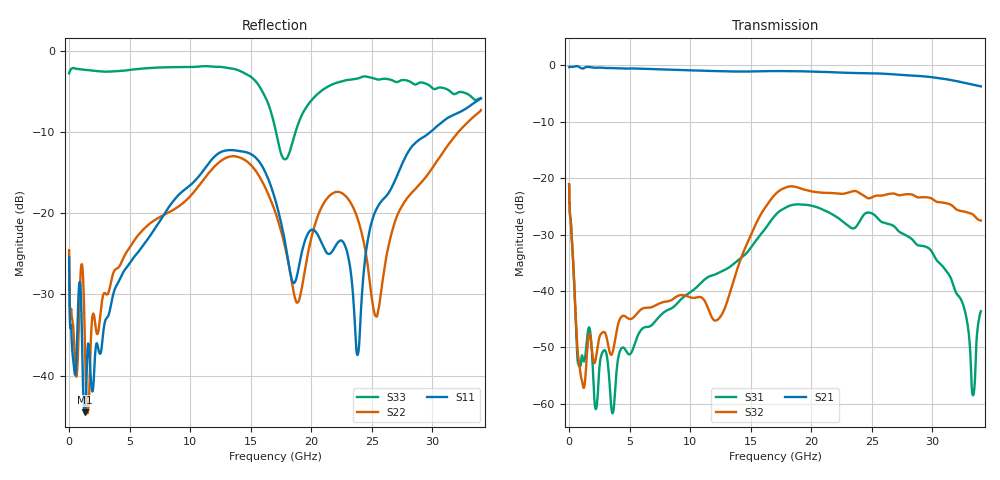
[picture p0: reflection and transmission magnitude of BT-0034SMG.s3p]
! MARKI MICROWAVE INC.
! Email:  info@markimicrowave.com  Phone:  408-778-4200
! Model Number:  BT-0034SM  Date:  01/13
! Filename:		BT_0034SM.S3P  Version: 1.0
! Description:  3-port S-parameter data for Bias Tee BT-0034SM
! Frequency Range: 	10 MHz to 34 GHz
! Port Configuration:	PORT 1: RF & DC
!  PORT 2: RF
!  Port 3: DC
! S3P File: Measurements: Mag<S11> Ang<S11> Mag<S12> Ang<S12> Mag<S13> Ang<S13> ! row 1
!  Mag<S21> Ang<S21> Mag<S22> Ang<S22> Mag<S23> Ang<S23> ! row 2
!  Mag<S31> Ang<S31> Mag<S32> Ang<S32> Mag<S33> Ang<S33> ! row 3
# GHz S  dB  R 50
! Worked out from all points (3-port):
!   801 points, 10 MHz to 34 GHz, reference 50 ohm
!   strongest paths, dB at 10 MHz, 8.51 GHz, 17.01 GHz, 25.51 GHz, 34 GHz:
!     S21: -0.3, -0.8, -1.0, -1.4, -3.7
!     S32: -21.0, -41.5, -22.9, -23.1, -27.5
!     S31: -21.1, -43.0, -26.6, -27.2, -43.6
!   lowest |S11| = -44.5 dB at 1.285 GHz (marker M1), VSWR 1.01, Z = 50.2 - j0.561 ohm
!   |S11| at or under -10 dB: start of sweep to 29.83 GHz
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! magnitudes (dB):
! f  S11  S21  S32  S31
! 10 MHz  -25.4  -0.3  -21.0  -21.1
! 1.285 GHz  -44.5  -0.4  -56.7  -52.3
! 3.623 GHz  -30.1  -0.5  -50.7  -61.6
! 11.91 GHz  -13.2  -1.0  -45.0  -37.2
! 17.01 GHz  -18.2  -1.0  -22.9  -26.6
! 23.81 GHz  -37.5  -1.4  -22.4  -28.3
! 25.38 GHz  -19.5  -1.4  -23.1  -26.9
! 31.2 GHz  -8.3  -2.5  -24.5  -36.6
! 33.37 GHz  -6.5  -3.4  -26.5  -58.5
! 34 GHz  -5.8  -3.7  -27.5  -43.6
